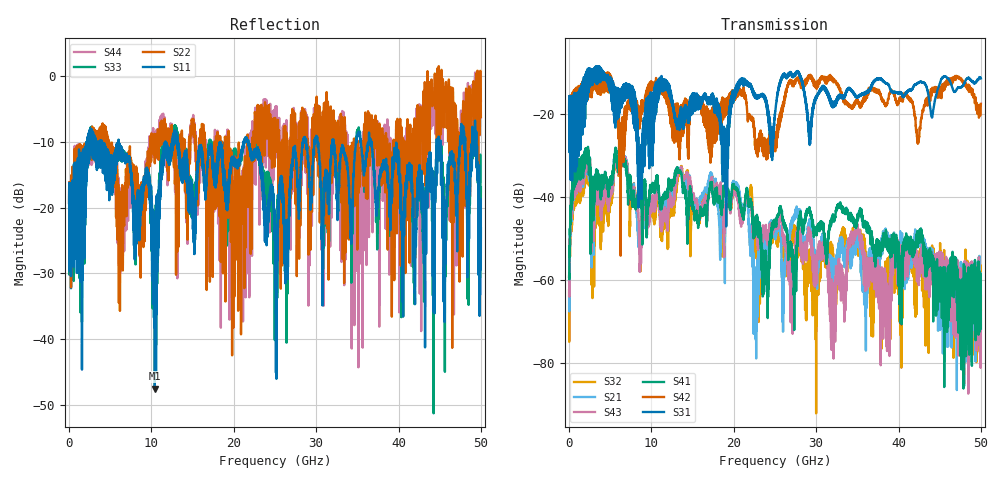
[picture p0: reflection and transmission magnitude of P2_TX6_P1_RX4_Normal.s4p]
!Keysight Technologies,N5225B,MY57041031,A.13.20.10
!Date: Friday, May 31, 2019 11:20:09
!Correction: S11(Full 4 Port(1,2,3,4))
!S12(Full 4 Port(1,2,3,4))
!S13(Full 4 Port(1,2,3,4))
!S14(Full 4 Port(1,2,3,4))
!S21(Full 4 Port(1,2,3,4))
!S22(Full 4 Port(1,2,3,4))
!S23(Full 4 Port(1,2,3,4))
!S24(Full 4 Port(1,2,3,4))
!S31(Full 4 Port(1,2,3,4))
!S32(Full 4 Port(1,2,3,4))
!S33(Full 4 Port(1,2,3,4))
!S34(Full 4 Port(1,2,3,4))
!S41(Full 4 Port(1,2,3,4))
!S42(Full 4 Port(1,2,3,4))
!S43(Full 4 Port(1,2,3,4))
!S44(Full 4 Port(1,2,3,4))
!S4P File: Measurements: <S11,S12,S13,S14>,
!<S21,S22,S23,S24>,
!<S31,S32,S33,S34>,
!<S41,S42,S43,S44>:
# Hz S  dB  R 50.0
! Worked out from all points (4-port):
!   5000 points, 10 MHz to 50 GHz, reference 50 ohm
!   strongest paths, dB at 10 MHz, 12.51 GHz, 25.01 GHz, 37.51 GHz, 50 GHz:
!     S31: -19.3, -16.8, -19.9, -11.6, -11.4
!     S42: -19.4, -19.5, -26.1, -14.8, -17.5
!     S41: -59.3, -36.9, -46.5, -51.7, -71.8
!     S43: -59.3, -41.5, -47.7, -63.4, -67.5
!     S21: -60.2, -38.9, -49.5, -54.6, -64.0
!     S32: -62.5, -43.6, -48.4, -56.8, -67.1
!   lowest |S11| = -47.5 dB at 10.41 GHz (marker M1), VSWR 1.01, Z = 50 - j0.419 ohm
!   |S11| at or under -10 dB: 13.21 GHz to 21.18 GHz (7.966 GHz wide, 46.3 % of centre); 21.74 GHz to 28.38 GHz (6.639 GHz wide, 26.5 % of centre); 36.67 GHz to 44.63 GHz (7.959 GHz wide, 19.6 % of centre)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
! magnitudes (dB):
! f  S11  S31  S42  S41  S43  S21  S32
! 10 MHz  -19.3  -19.3  -19.4  -59.3  -59.3  -60.2  -62.5
! 2.15 GHz  -14.6  -16.8  -16.0  -29.7  -30.5  -30.8  -31.5
! 10.41 GHz  -47.5  -14.8  -12.3  -38.8  -43.2  -42.8  -45.9
! 12.86 GHz  -8.3  -20.3  -19.4  -34.9  -38.3  -36.9  -41.2
! 22.65 GHz  -12.3  -15.3  -27.0  -47.0  -46.0  -58.4  -52.5
! 27.84 GHz  -19.9  -10.2  -11.3  -46.8  -48.0  -43.4  -52.9
! 50 GHz  -23.1  -11.4  -17.5  -71.8  -67.5  -64.0  -67.1
